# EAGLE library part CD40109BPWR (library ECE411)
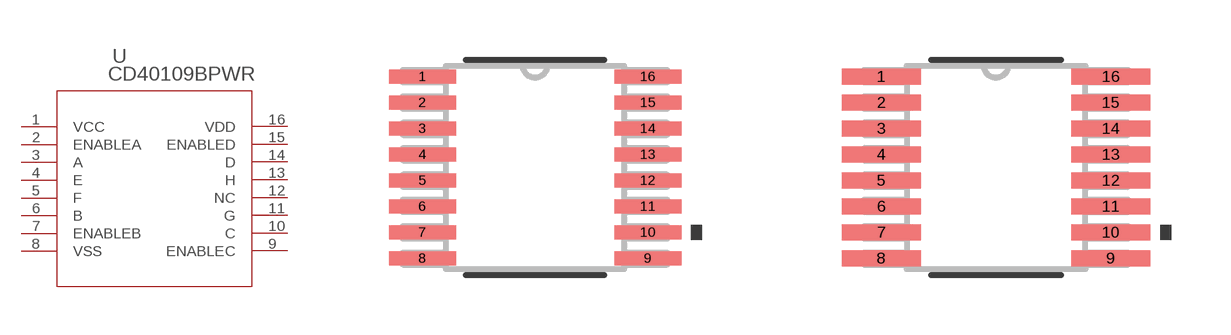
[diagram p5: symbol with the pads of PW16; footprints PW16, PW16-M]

Designator prefix U

## CD40109BPWR (MANUFACTURER_PART_NUMBER: CD40109BPWR; VENDOR: Vendor)  [PW16]
1  VCC  pwr
2  ENABLEA  in
3  A  in
4  E  out
5  F  out
6  B  in
7  ENABLEB  in
8  VSS  pwr
9  ENABLEC  in
10  C  in
11  G  out
12  NC  nc
13  H  out
14  D  in
15  ENABLED  in
16  VDD  pwr

## CD40109BPWRPW16-M (MANUFACTURER_PART_NUMBER: CD40109BPWR; VENDOR: Vendor)  [PW16-M]
Pads as for PW16

## CD40109BPWRPW16-L (MANUFACTURER_PART_NUMBER: CD40109BPWR; VENDOR: Vendor)  [PW16-L]
Pads as for PW16

## Footprint PW16 (pad centres in mm)
smd 1.676 x 0.356: 1 -2.819,2.275; 2 -2.819,1.625; 3 -2.819,0.975; 4 -2.819,0.325; 5 -2.819,-0.325; 6 -2.819,-0.975; 7 -2.819,-1.625; 8 -2.819,-2.275; 9 2.819,-2.275; 10 2.819,-1.625; 11 2.819,-0.975; 12 2.819,-0.325; 13 2.819,0.325; 14 2.819,0.975; 15 2.819,1.625; 16 2.819,2.275

## Footprint PW16-M (pad centres in mm)
smd 1.981 x 0.406: 1 -2.87,2.275; 2 -2.87,1.625; 3 -2.87,0.975; 4 -2.87,0.325; 5 -2.87,-0.325; 6 -2.87,-0.975; 7 -2.87,-1.625; 8 -2.87,-2.275; 9 2.87,-2.275; 10 2.87,-1.625; 11 2.87,-0.975; 12 2.87,-0.325; 13 2.87,0.325; 14 2.87,0.975; 15 2.87,1.625; 16 2.87,2.275

## Footprint PW16-L (pad centres in mm)
smd 1.372 x 0.305: 1 -2.769,2.275; 2 -2.769,1.625; 3 -2.769,0.975; 4 -2.769,0.325; 5 -2.769,-0.325; 6 -2.769,-0.975; 7 -2.769,-1.625; 8 -2.769,-2.275; 9 2.769,-2.275; 10 2.769,-1.625; 11 2.769,-0.975; 12 2.769,-0.325; 13 2.769,0.325; 14 2.769,0.975; 15 2.769,1.625; 16 2.769,2.275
